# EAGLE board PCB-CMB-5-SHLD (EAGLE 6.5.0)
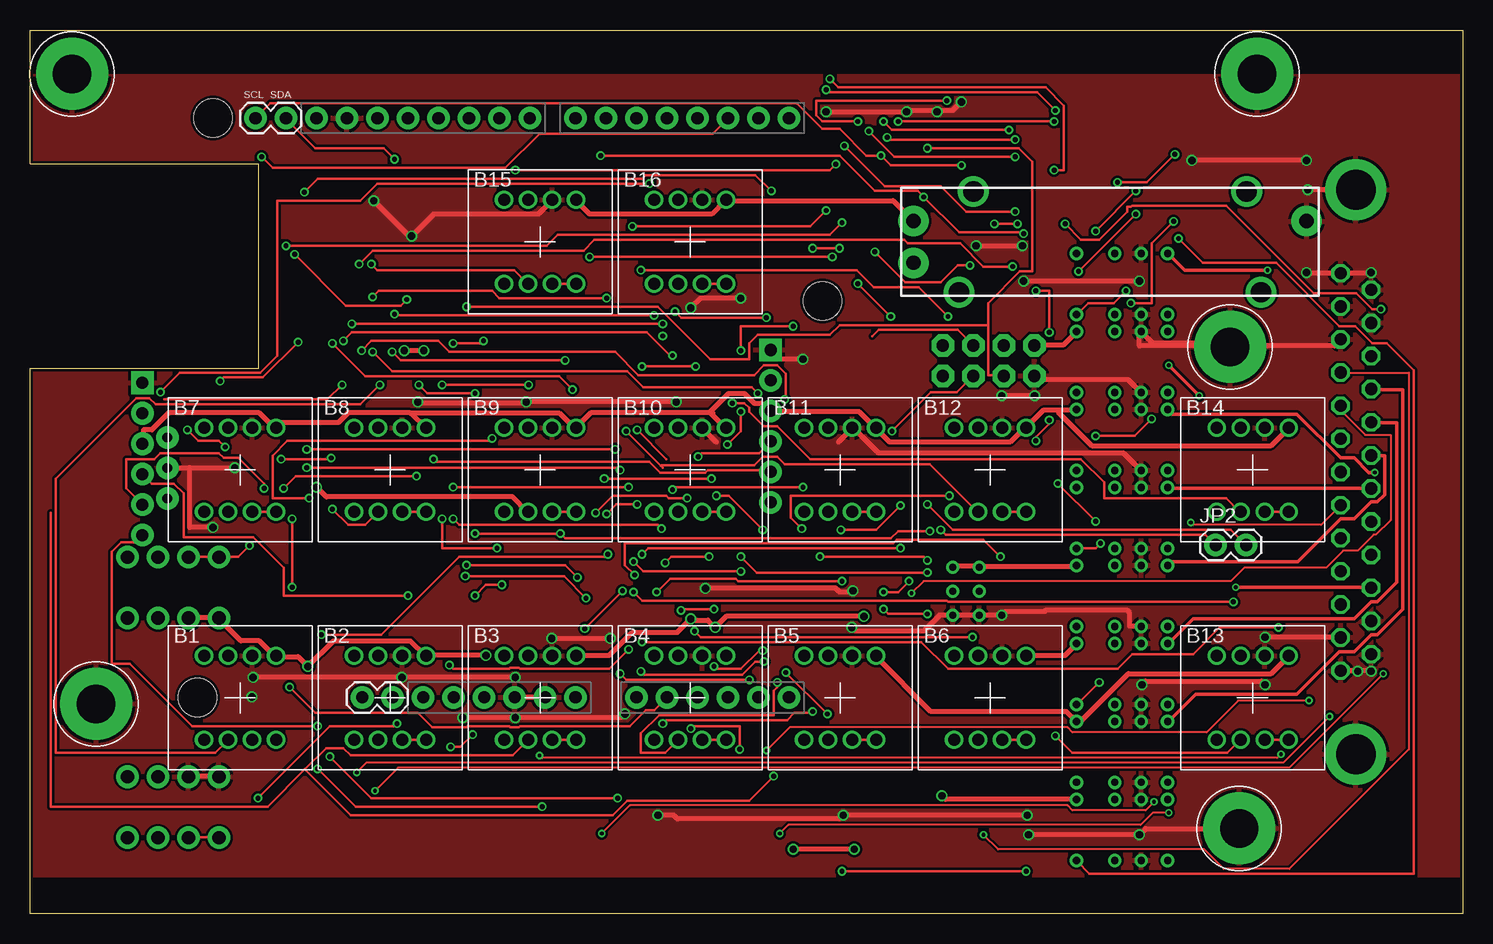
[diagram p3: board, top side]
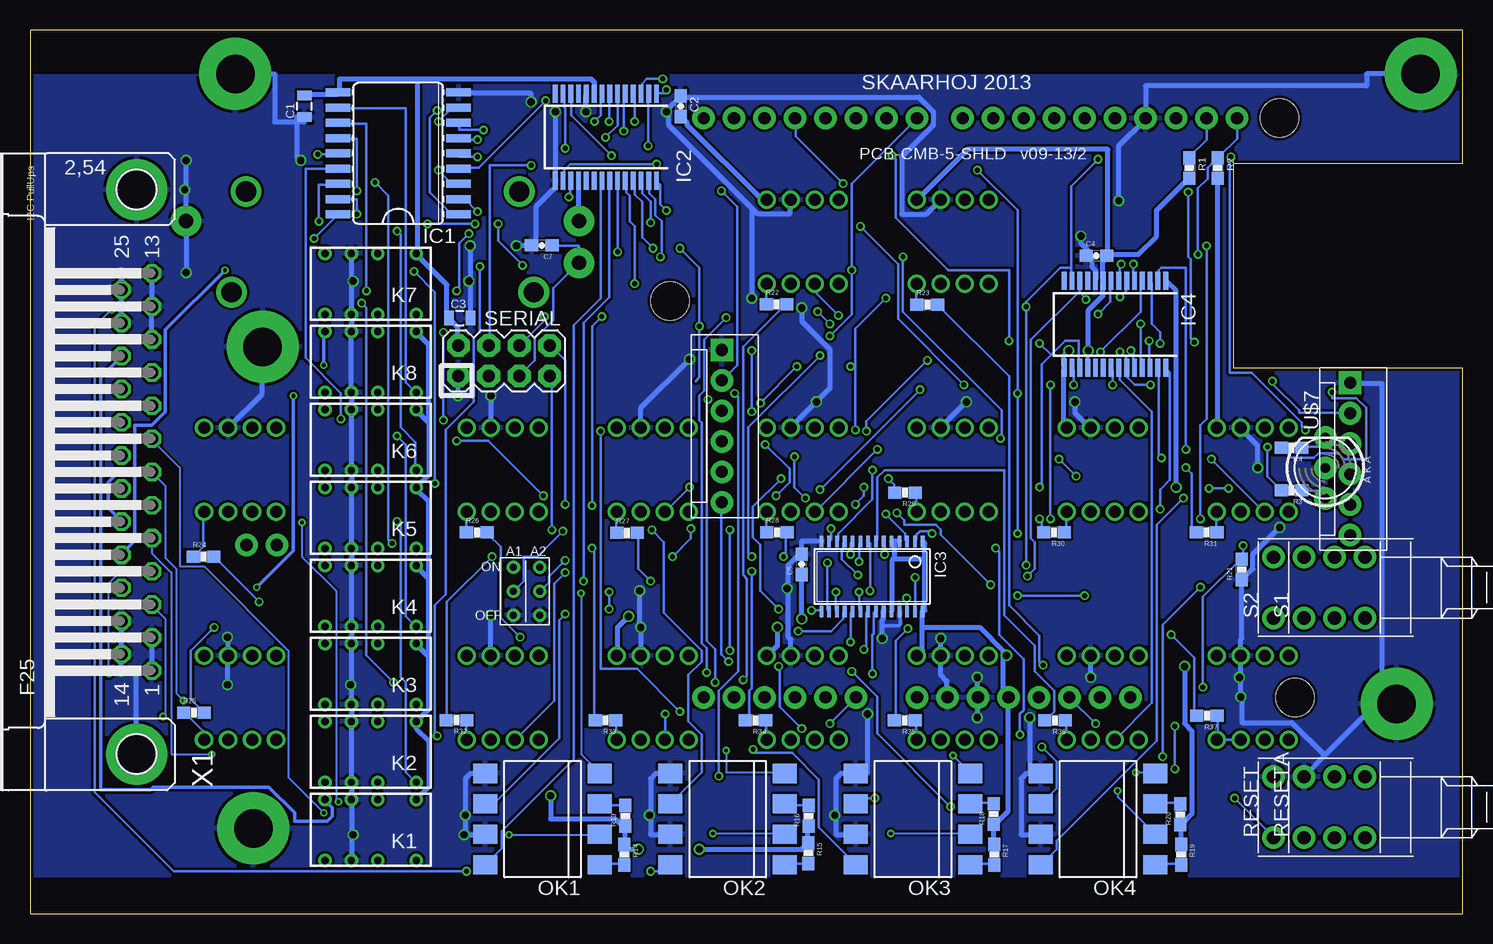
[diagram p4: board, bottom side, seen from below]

Size 119.38 x 73.66 mm. Coordinates in mm from the lower left corner, seen from the top.
Outline: 0,0 0,45.47 19.05,45.47 19.05,62.5 0,62.5 0,73.66 119.38,73.66 119.38,0 0,0
Copper layers (1*16): Top 0.035mm / dielectric 1.5mm / Bottom 0.035mm
Design rules "Fusion_eagle_rule_v1.1": minimum track width 6mil, minimum drill 12mil, track to track 6mil, track to pad 6mil, pad to pad 6mil, via to via 6mil, smd to smd 0mil, copper to edge 10mil, drill to drill 10mil, minimum pad ring 10mil, minimum via ring 6mil, stop-mask expansion 2mil, vias tented up to drill 100mil, thermal gap 10mil
Net classes: 0 default: width 0.203 mm, drill 0.406 mm, clearance 0.203 mm; 1 PWR: width 0.406 mm, drill 0.61 mm, clearance 0.203 mm; 2 RELAY LINES: width 0.305 mm, clearance 0.203 mm; 3 INput lines: clearance 0.203 mm
Holes 3.2 mm at 66.04,51.07 15.24,66.31 13.97,18.05
tRestrict: area 0,0 to 120,3; area 0,70 to 120,74
bRestrict: area 0,70 to 120,74; area 0,0 to 120,3

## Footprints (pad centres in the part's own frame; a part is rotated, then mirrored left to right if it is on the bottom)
NKK-NP01 = drill 1: 1 1,3.5; 2 -1,-3.5; L1 3,-3.5; L2 1,-3.5; L3 -1,3.5; L4 -3,3.5; LC1 3,3.5; LC2 -3,-3.5
0805 = smd 0.8 x 1.2: 1 -0.9,0; 2 0.9,0
0603-CAP = smd 1.1 x 1: 1 -0.85,0; 2 0.85,0
DUEMILANOVE_VIAS = drill 1.016 pad 1.88: 3.3V 50.8,13.97; 5V 50.8,16.51; A0 50.8,29.21; A1 50.8,31.75; A2 50.8,34.29; A3 50.8,36.83; A4 50.8,39.37; A5 50.8,41.91; AREF 2.54,2.54; D2 2.54,36.83; D3 2.54,34.29; D4 2.54,31.75; D5 2.54,29.21; D6 2.54,26.67; D7 2.54,24.13; D8 2.54,20.32; D9 2.54,17.78; D10 2.54,15.24; D11 2.54,12.7; D12 2.54,10.16; D13 2.54,7.62; GND@0 50.8,19.05; GND@1 50.8,21.59; GND@2 2.54,5.08; RES 50.8,11.43; RX 2.54,41.91; TX 2.54,39.37; VIN 50.8,24.13
SO18W = smd 0.66 x 2.032: 1 -5.08,-5.029; 2 -3.81,-5.029; 3 -2.54,-5.029; 4 -1.27,-5.029; 5 0,-5.029; 6 1.27,-5.029; 7 2.54,-5.029; 8 3.81,-5.029; 9 5.08,-5.029; 10 5.08,5.029; 11 3.81,5.029; 12 2.54,5.029; 13 1.27,5.029; 14 0,5.029; 15 -1.27,5.029; 16 -2.54,5.029; 17 -3.81,5.029; 18 -5.08,5.029
SSOP28 = smd 0.4 x 1.5: 1 -4.225,-3.625; 2 -3.575,-3.625; 3 -2.925,-3.625; 4 -2.275,-3.625; 5 -1.625,-3.625; 6 -0.975,-3.625; 7 -0.325,-3.625; 8 0.325,-3.625; 9 0.975,-3.625; 10 1.625,-3.625; 11 2.275,-3.625; 12 2.925,-3.625; 13 3.575,-3.625; 14 4.225,-3.625; 15 4.225,3.625; 16 3.575,3.625; 17 2.925,3.625; 18 2.275,3.625; 19 1.625,3.625; 20 0.975,3.625; 21 0.325,3.625; 22 -0.325,3.625; 23 -0.975,3.625; 24 -1.625,3.625; 25 -2.275,3.625; 26 -2.925,3.625; 27 -3.575,3.625; 28 -4.225,3.625
TSSOP28 = smd 0.305 x 0.991: 1 -4.225,-2.918; 2 -3.575,-2.918; 3 -2.925,-2.918; 4 -2.275,-2.918; 5 -1.625,-2.918; 6 -0.975,-2.918; 7 -0.325,-2.918; 8 0.325,-2.918; 9 0.975,-2.918; 10 1.625,-2.918; 11 2.275,-2.918; 12 2.925,-2.918; 13 3.575,-2.918; 14 4.225,-2.918; 15 4.225,2.918; 16 3.575,2.918; 17 2.925,2.918; 18 2.275,2.918; 19 1.625,2.918; 20 0.975,2.918; 21 0.325,2.918; 22 -0.325,2.918; 23 -0.975,2.918; 24 -1.625,2.918; 25 -2.275,2.918; 26 -2.925,2.918; 27 -3.575,2.918; 28 -4.225,2.918
1X02 = drill 1.016 pad 1.88: 1 0,0; 2 2.54,0
MOLEX-1X6 = drill 1.016 pad 1.88 square: 1 0,0 | drill 1.016 pad 1.88: 2 2.54,0; 3 5.08,0; 4 7.62,0; 5 10.16,0; 6 12.7,0
DS2Y = drill 0.6: 1 1.2,0.46; 16 1.2,5.54; O1 4.4,0.46; O2 4.4,5.54; P1 6.6,0.46; P2 6.6,5.54; S1 8.8,0.46; S2 8.8,5.54
DIL8-SMD = smd 1.6 x 2: 1 -3.81,-4.77; 2 -1.27,-4.77; 3 1.27,-4.77; 4 3.81,-4.77; 5 3.81,4.77; 6 1.27,4.77; 7 -1.27,4.77; 8 -3.81,4.77
SLIDER20 = drill 1.194 pad 2.54: 1 -16.383,1.74; 2A -16.383,-1.74; 3 16.383,1.74 | drill 1.702: P$1 -11.392,4.191; P$2 11.392,4.191; P$3 12.598,-4.191; P$4 -12.598,-4.191
0603-RES = smd 1.1 x 1: 1 -0.85,0; 2 0.85,0
PUSHBUTTON = drill 1.1 pad 1.88: 1 2.54,2.54; 2 2.54,-2.54; 3 -2.54,2.54; 4 -2.54,-2.54
2X4 = drill 1.016 pad 1.88 octagon: 1 -3.81,-1.27; 2 -3.81,1.27; 3 -1.27,-1.27; 4 -1.27,1.27; 5 1.27,-1.27; 6 1.27,1.27; 7 3.81,-1.27; 8 3.81,1.27
3.2MMPAD6MM = drill 3.2 pad 6: P$1 0,0
LED5MM-BICOLOR = drill 0.813 pad 1.88: A2 2.54,0; A3 -2.54,0; K1 0,0
2BITADDR = drill 0.6: A1 0,0; A2 2.2,0; H2 0,2; H3 2.2,2; L2 0,-2; L3 2.2,-2
F25HP = drill 1.016 octagon: 1 -16.561,-1.27; 2 -13.792,-1.27; 3 -11.049,-1.27; 4 -8.28,-1.27; 5 -5.512,-1.27; 6 -2.769,-1.27; 7 0,-1.27; 8 2.769,-1.27; 9 5.512,-1.27; 10 8.28,-1.27; 11 11.049,-1.27; 12 13.792,-1.27; 13 16.561,-1.27; 14 -15.189,1.27; 15 -12.421,1.27; 16 -9.652,1.27; 17 -6.909,1.27; 18 -4.14,1.27; 19 -1.372,1.27; 20 1.372,1.27; 21 4.14,1.27; 22 6.909,1.27; 23 9.652,1.27; 24 12.421,1.27; 25 15.189,1.27 | drill 3.302 pad 5.08: G1 -23.52,0; G2 23.52,0

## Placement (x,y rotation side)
B1  NKK-NP01-SINGLECOLOR  [NKK-NP01]  17.5,18 0 top
B2  NKK-NP01-SINGLECOLOR  [NKK-NP01]  30,18 0 top
B3  NKK-NP01-SINGLECOLOR  [NKK-NP01]  42.5,18 0 top
B4  NKK-NP01-SINGLECOLOR  [NKK-NP01]  55,18 0 top
B5  NKK-NP01-SINGLECOLOR  [NKK-NP01]  67.5,18 0 top
B6  NKK-NP01-SINGLECOLOR  [NKK-NP01]  80,18 0 top
B7  NKK-NP01-SINGLECOLOR  [NKK-NP01]  17.5,37 0 top
B8  NKK-NP01-SINGLECOLOR  [NKK-NP01]  30,37 0 top
B9  NKK-NP01-SINGLECOLOR  [NKK-NP01]  42.5,37 0 top
B10  NKK-NP01-SINGLECOLOR  [NKK-NP01]  55,37 0 top
B11  NKK-NP01-SINGLECOLOR  [NKK-NP01]  67.5,37 0 top
B12  NKK-NP01-SINGLECOLOR  [NKK-NP01]  80,37 0 top
B13  NKK-NP01-SINGLECOLOR  [NKK-NP01]  101.88,18 0 top
B14  NKK-NP01-SINGLECOLOR  [NKK-NP01]  101.88,37 0 top
B15  NKK-NP01-SINGLECOLOR  [NKK-NP01]  42.5,56 0 top
B16  NKK-NP01-SINGLECOLOR  [NKK-NP01]  55,56 0 top
C1  100nF  [0805]  96.52,67.31 90 bottom
C2  100nF  [0603-CAP]  65.15,67.31 270 bottom
C3  10uF  [0805]  83.57,49.66 0 bottom
C4  100nF  [0603-CAP]  30.51,54.86 0 bottom
C5  100nF  [0603-CAP]  55.07,29.13 90 bottom
C7  10nF  [0603-CAP]  76.73,55.71 180 bottom
GND  ARDUINO_SHIELDNO_SILK  [DUEMILANOVE_VIAS]  21.34,68.85 270 top
IC1  ULN2803A  [SO18W]  88.7,63.38 90 bottom
IC2  MCP23017SS  [SSOP28]  71.39,64.73 180 bottom
IC3  PCA9685  [TSSOP28]  49.21,28.12 180 bottom
IC4  MCP23017SS  [SSOP28]  28.97,49.12 180 bottom
JP1  [1X02]  27.69,18.05 0 top
JP2  [1X02]  98.81,30.75 0 top
JP3  [MOLEX-1X6]  61.72,47 270 bottom
JP4  [1X02]  21.34,66.31 180 top
JP5  [MOLEX-1X6]  9.36,44.26 270 bottom
K1  RELAY5VIM03  [DS2Y]  86,10 180 bottom
K2  RELAY5VIM03  [DS2Y]  86,16.5 180 bottom
K3  RELAY5VIM03  [DS2Y]  86,23 180 bottom
K4  RELAY5VIM03  [DS2Y]  86,29.5 180 bottom
K5  RELAY5VIM03  [DS2Y]  86,36 180 bottom
K6  RELAY5VIM03  [DS2Y]  86,42.5 180 bottom
K7  RELAY5VIM03  [DS2Y]  86,55.5 180 bottom
K8  RELAY5VIM03  [DS2Y]  86,49 180 bottom
OK1  LTV826S  [DIL8-SMD]  76.67,7.9 90 bottom
OK2  LTV826S  [DIL8-SMD]  61.24,7.9 90 bottom
OK3  LTV826S  [DIL8-SMD]  45.81,7.9 90 bottom
OK4  LTV826S  [DIL8-SMD]  30.38,7.9 90 bottom
POT1  10K Linear  [SLIDER20]  90,56 0 top
R1  1K5  [0603-RES]  22.77,62.15 270 bottom
R2  1K5  [0603-RES]  20.4,62.15 270 bottom
R3  270  [0603-RES]  14.24,35.29 180 bottom
R4  270  [0603-RES]  14.24,38.83 180 bottom
R13  330R  [0603-RES]  69.76,8.18 90 bottom
R14  330R  [0603-RES]  69.86,4.93 270 bottom
R15  330R  [0603-RES]  54.53,5.06 270 bottom
R16  330R  [0603-RES]  54.47,8.18 90 bottom
R17  330R  [0603-RES]  39.03,4.93 270 bottom
R18  330R  [0603-RES]  39.06,8.32 90 bottom
R19  330R  [0603-RES]  23.46,4.93 270 bottom
R20  330R  [0603-RES]  23.52,8.3 90 bottom
R21  10K  [0603-RES]  18.41,28.72 90 bottom
R22  100R  [0603-RES]  57.16,50.8 0 bottom
R23  100R  [0603-RES]  44.61,50.77 0 bottom
R24  100R  [0603-RES]  104.91,29.77 0 bottom
R25  100R  [0603-RES]  105.72,16.77 0 bottom
R26  100R  [0603-RES]  82.15,31.79 0 bottom
R27  100R  [0603-RES]  69.62,31.75 0 bottom
R28  100R  [0603-RES]  57.14,31.82 0 bottom
R29  100R  [0603-RES]  46.47,35.11 180 bottom
R30  100R  [0603-RES]  34.04,31.8 180 bottom
R31  100R  [0603-RES]  21.32,31.8 180 bottom
R32  100R  [0603-RES]  83.84,16.16 180 bottom
R33  100R  [0603-RES]  71.41,16.14 180 bottom
R34  100R  [0603-RES]  58.93,16.12 180 bottom
R35  100R  [0603-RES]  46.48,16.12 180 bottom
R36  100R  [0603-RES]  33.96,16.12 180 bottom
R37  100R  [0603-RES]  21.31,16.5 180 bottom
RESET  [PUSHBUTTON]  13.21,8.89 90 bottom
RESETA  [PUSHBUTTON]  10.67,8.89 90 bottom
S1  [PUSHBUTTON]  10.67,27.19 90 bottom
S2  [PUSHBUTTON]  13.21,27.19 90 bottom
SERIAL  M04X2  [2X4]  79.88,46.1 0 bottom
U$4  GNDPAD6MM  [3.2MMPAD6MM]  100,47.25 0 top
U$7  LEDBICOLOR-AKA  [LED5MM-BICOLOR]  11.44,37.16 90 bottom
U$15  GNDPAD6MM  [3.2MMPAD6MM]  100.77,7.12 0 top
U$18  GNDPAD6MM  [3.2MMPAD6MM]  102.26,70 0 top
U$19  2BITADDR  [2BITADDR]  79.1,26.89 0 bottom
U$20  GNDPAD6MM  [3.2MMPAD6MM]  5.5,17.5 0 top
U$21  GNDPAD6MM  [3.2MMPAD6MM]  3.5,70 0 top
X1  DB25F  [F25HP]  110.49,36.83 90 bottom

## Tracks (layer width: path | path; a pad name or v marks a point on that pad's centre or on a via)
5V  (via drill 0.61)
  Top 0.406: B15.LC1 45.52,59.44 46.63,58.32 56.79,58.32 57.91,59.44 B16.LC1 58.12,59.44 71.93,59.44 73.56,57.81 POT1.1 | 56.69,41.76 46.74,41.76 45.52,40.54 B9.LC1 45.31,40.54 44.09,41.76 31.9,41.76 31.8,41.66 | 56.79,41.66 57.91,40.54 B10.LC1 | 56.79,41.66 56.69,41.76 | 56.9,41.76 56.79,41.66 | v32.82,46.94 v31.19,46.94 | 31.8,41.66 32.92,40.54 B8.LC1 | 31.8,41.66 31.7,41.76 26.52,41.76 25.7,40.95 20.93,40.95 20.52,40.54 B7.LC1 20.32,40.54 19.1,41.76 11.58,41.76 10.16,40.34 9.45,40.34 9.45,39.22 JP5.3 | S1.3 13.21,24.69 15.75,24.69 S2.3 15.85,24.49 17.58,22.76 19.1,22.76 20.32,21.54 B1.LC1 20.52,21.44 22.35,21.44 v23.16,20.62 25.3,22.76 31.7,22.76 32.92,21.54 B2.LC1 33.12,21.54 v38,21.54 | B3.LC1 45.52,21.54 48.26,21.54 50.19,23.47 53.95,23.47 v55.07,24.59 55.17,24.49 56.49,24.49 v57.1,23.88 58.01,24.79 v69.49,24.79 | K8.1 87.17,48.46 86.16,47.45 83.72,47.45 SERIAL.2 | 85.65,41.96 87.17,41.96 K6.1 | 85.65,41.96 84.43,41.96 83.01,40.54 B12.LC1 82.8,40.44 81.69,39.32 71.63,39.32 70.61,40.34 B11.LC1 70.41,40.54 69.09,41.86 61.77,41.86 JP3.3 61.57,41.96 60.96,42.57 60.35,42.57 59.54,43.38 58.22,43.38 56.69,41.86 56.69,41.76 | B14.LC1 104.85,40.44 103.43,39.01 88.49,39.01 85.65,41.86 85.65,41.96 | v68.68,5.38 v63.6,5.38 | U$19.H3 76.91,28.96 79.05,28.96 U$19.H2 79.25,28.96 87.17,28.96 K4.1 | K3.1 87.17,22.45 86.26,21.54 83.01,21.54 B6.LC1 | B5.LC1 70.51,21.44 75.08,16.87 86.36,16.87 87.17,16.05 K2.1 87.38,16.05 87.58,16.05 91.54,20.02 103.43,20.02 104.85,21.44 B13.LC1 | v76,9.86 76.3,9.55 87.17,9.55 K1.1
  Bottom 0.305: v31.19,46.94 31.25,46.94 IC4.18
  Bottom 0.406: IC2.18 73.66,61.06 73.66,57.81 POT1.1 | C2.2 65.13,66.45 64.62,65.94 64.62,65.73 58.42,59.54 58.01,59.54 B16.LC1 | R2.2 20.42,61.27 20.42,40.54 B7.LC1 | R1.2 22.86,61.27 25.5,58.62 25.5,56.49 27.03,54.97 29.57,54.97 29.57,54.86 C4.2 | B8.LC1 33.02,40.54 33.22,40.74 33.22,45.41 IC4.15 33.22,45.62 33.22,46.53 v32.82,46.94 | v31.19,46.94 31.19,50.29 29.97,51.51 29.97,52.73 IC4.9 29.97,52.93 29.97,54.36 29.67,54.66 C4.2 | B15.LC1 45.41,59.54 41.25,63.7 29.57,63.7 29.57,55.07 C4.2 | R19.1 23.47,5.79 23.47,7.42 R20.1 23.37,7.52 22.55,8.33 22.55,15.24 23.16,15.85 v23.16,20.62 | R17.1 39.12,5.79 39.12,7.42 R18.1 38.91,7.52 37.9,8.53 37.9,17.98 GND.5V 37.9,18.19 38.3,18.59 38.3,21.54 | 47.35,31.09 47.55,31.09 IC3.5 | 47.35,31.09 46.94,31.09 IC3.4 | 47.35,29.67 47.55,29.46 47.55,25.3 IC3.24 | 47.35,31.09 47.35,29.67 | 45.01,23.88 45.01,21.95 45.41,21.54 B3.LC1 | 45.01,23.88 45.01,25.2 IC3.28 44.81,25.3 44.81,29.57 | 44.81,29.57 44.81,30.89 44.91,30.99 IC3.1 | v55.07,24.59 55.07,28.25 C5.1 | v57.1,23.88 57.1,22.35 57.91,21.54 B4.LC1 | 44.81,29.57 47.24,29.57 47.35,29.67 | 38.3,21.54 38.3,21.95 40.23,23.88 45.01,23.88 | 38.3,21.54 v38,21.54 | C1.2 96.52,68.28 93.78,68.28 93.78,68.38 IC1.10 93.57,68.58 93.57,69.6 87.07,69.6 | 87.07,69.6 72.64,69.6 72.34,69.29 72.34,68.38 IC2.9 | SERIAL.2 83.72,47.45 83.72,48.87 84.43,49.58 C3.1 84.63,49.78 84.63,52.43 87.17,54.97 K7.1 87.07,55.17 87.07,69.6 | 86.26,41.05 87.17,41.96 K6.1 | 86.26,41.05 86.16,40.95 86.16,36.58 87.17,35.56 K5.1 87.17,35.36 86.16,34.34 86.16,28.14 86.26,28.04 | K8.1 87.17,48.46 86.16,47.45 86.16,41.15 86.26,41.05
  Bottom 0.406: R16.1 54.56,7.32 54.56,5.99 R15.1 54.66,5.79 55.07,5.38 v63.6,5.38 | v68.68,5.38 69.6,5.38 69.6,5.79 R14.1 69.8,5.79 69.8,7.32 R13.1 70,7.32 70.61,7.92 76,7.92 v76,9.86 | K1.1 87.17,9.55 86.16,10.57 86.16,14.43 87.17,15.44 87.17,15.95 K2.1 87.07,16.15 86.16,17.07 86.16,21.44 86.26,21.54 | 86.26,21.54 87.17,22.45 K3.1 | 86.26,28.04 86.16,27.94 86.16,21.64 86.26,21.54 | 86.26,28.04 87.17,28.96 K4.1 | v69.49,24.79 70.41,23.88 70.41,21.54 B5.LC1
A1  (via drill 0.41)
  Top 0.203: v74.98,31.9 72.34,31.9 71.73,31.29 44.6,31.29 v44.2,31.7 v37.08,31.7 | v32.41,44.09 33.12,43.38 v37.08,43.38 | v67.16,62.48 66.65,61.98 v40.44,61.98
  Bottom 0.203: v44.2,31.7 44.2,31.9 45.21,31.9 45.52,31.6 45.52,31.19 45.62,31.09 IC3.2 | v74.98,31.9 77.11,29.77 78.23,29.77 78.23,27.74 79.05,26.92 U$19.A1 | v32.41,44.09 32.41,45.31 32.51,45.41 IC4.16 | v37.08,31.7 v37.08,43.38 37.08,58.62 v40.44,61.98 | v67.16,62.48 74.37,62.48 74.88,61.98 74.88,61.16 IC2.16
A1CFG  (via drill 0.41)
  Top 0.203: v18.29,30.68 17.37,29.77 15.75,29.77 | v21.64,18.9 23.77,16.76 32.31,16.76 33.53,15.54 36.37,15.54 36.47,15.65 39.93,15.65 40.03,15.54 40.74,15.54 40.84,15.65 49.99,15.65 51.31,16.97 52.02,16.97 53.03,17.98 GND.A1 | 15.75,29.77 13.21,29.77 S1.1 | 15.75,29.77 S2.1
  Bottom 0.203: v18.29,30.68 18.29,29.77 18.39,29.67 R21.2 18.49,29.57 21.64,26.42 v21.64,18.9
A2  (via drill 0.41)
  Top 0.203: v48.06,33.33 48.87,34.14 v50.6,34.14 | v35.26,35.56 v49.89,35.56 | v47.55,63.2 67.46,63.2 70.41,60.25 73.97,60.25 v74.47,59.74 77.42,56.79 82.7,56.79 v82.8,56.69 | v37.8,47.75 37.59,47.55 v35.26,47.55 | v74.78,29.46 74.47,29.77 v65.84,29.77 | v64.31,32.11 63.4,33.02 63.4,34.85 v76.61,34.85 | v83.82,39.42 83.82,39.73 84.94,40.84 v84.94,41.15 | v84.94,48.46 84.94,51.92 v83.82,51.92
  Bottom 0.203: v48.06,33.33 46.43,31.7 46.43,31.19 46.33,31.09 IC3.3 | v50.6,34.14 49.89,34.85 v49.89,35.56 | v35.26,35.56 35.05,35.76 35.05,45.82 34.29,46.58 | 34.29,46.58 33.12,47.75 32,47.75 32,45.62 31.9,45.52 IC4.17 | v74.47,59.74 74.37,59.84 74.37,61.06 IC2.17 | v47.55,63.2 47.24,62.89 47.24,58.01 42.88,53.65 37.8,53.65 v37.8,47.75 | 34.29,46.58 v35.26,47.55 | v74.78,29.46 76.1,28.14 76.1,27.64 76.81,26.92 U$19.A2 | v65.84,29.77 64.31,31.29 v64.31,32.11 | v76.61,34.85 81.18,39.42 v83.82,39.42 | v84.94,48.46 v84.94,41.15 | v83.82,51.92 83.62,52.12 83.62,55.88 v82.8,56.69
D2  (via drill 0.41)
  Top 0.203: v16.26,38.91 15.75,39.42 14.02,39.42 v13.11,40.34 | v19.3,63.09 20.22,62.18 39.62,62.18 42.47,65.02 56.9,65.02 58.12,66.24 GND.D2
  Bottom 0.203: v16.26,38.91 16.26,36.47 15.14,35.36 R3.2 | v13.11,40.34 13.41,40.64 13.41,40.95 17.58,45.11 19.41,45.11 19.41,62.99 v19.3,63.09
D3  (via drill 0.41)
  Top 0.203: v10.87,43.48 12.5,45.11 19.2,45.11 20.62,46.53 20.62,59.44 27.53,59.44 28.96,60.86 v51.61,60.86
  Bottom 0.203: v10.87,43.48 10.87,42.98 8.84,42.98 8.03,42.16 8.03,37.9 9.86,37.9 10.36,38.41 11.99,38.41 12.39,38 14.22,38 15.04,38.81 R4.2 | v51.61,60.86 55.58,64.82 55.58,66.24 GND.D3
DISP_DATA_OUT  (via drill 0.41)
  Top 0.203: 70.21,48.16 70.71,48.67 77.32,48.67 78.54,47.45 SERIAL.6 | v76.5,49.78 74.07,52.22 70.31,52.22 68.89,53.65 v50.9,53.65
  Bottom 0.203: v52.73,48.16 50.9,49.99 v50.9,53.65 50.9,60.86 45.52,66.24 GND.D7 | v76.5,49.78 76.5,49.48 78.54,47.45 SERIAL.6
GND  (via drill 0.61)
  Top 0.406: RESETA.1 13.21,11.48 15.75,11.48 RESET.1 | v111.76,53.44 109.22,53.44 X1.13 109.12,53.44 v106.38,53.44 | v106.38,62.79 v96.83,62.79 | X1.G2 v106.48,60.35 | v68.48,23.88 68.78,23.57 74.47,23.57 75.79,24.89 76.71,24.89 U$19.L3 76.91,24.89 79.05,24.89 U$19.L2 79.25,24.89 v80.97,24.89 81.28,25.2 84.53,25.2 84.63,25.3 91.44,25.3 91.64,25.09 91.64,23.98 92.56,23.98 K4.P2 | v56.29,27.13 67.16,27.13 67.46,26.82 68.48,26.82 v68.58,26.92 | v78.84,55.68 v82.7,55.68 | v43.48,22.96 v48.36,22.96 | v40.44,19.71 v30.99,19.71 v18.59,19.71 | GND.GND@1 42.88,18.09 40.44,18.09 GND.GND@0 | v36.07,16.36 v40.44,16.36 49.28,16.36 v49.58,16.66 | v102.92,23.06 109.22,23.06 X1.2 | v111.76,20.22 111.66,20.32 110.64,20.32 | 110.64,20.32 109.22,20.32 X1.1 | v110.64,20.22 110.64,20.32 | v52.32,8.23 53.65,8.23 53.95,7.92 67.46,7.92 v67.77,8.23 v83.11,8.23 | v83.72,43.18 v80.97,43.18 | v83.21,6.6 v92.46,6.6 92.96,7.11 100.69,7.11 U$15.P$1 | v102.92,19.1 102.62,19.41 92.96,19.41 v92.66,19.1 | v92.46,52.73 v82.8,52.73 | v32.31,42.67 32.41,42.57 41.25,42.57 v41.35,42.67 v53.85,42.67 | 57.2,39.32 56.08,40.44 B10.1 | 67.36,39.32 68.48,40.44 B11.1 68.68,40.44 70.71,38.41 91.14,38.41 92.56,36.98 K6.P2 | B15.1 43.48,59.44 42.37,58.32 33.63,58.32 v31.8,56.49 31.7,56.59 31.5,56.59 v28.65,59.44 | v66.34,66.85 v73.05,66.85 73.15,66.95 75.59,66.95 | v77.62,67.67 76.91,66.95 75.59,66.95 | v75.59,66.85 75.59,66.95 | v64.41,46.23 62.48,46.23 61.77,46.94 JP3.1 | v55.07,50.49 55.88,51.31 v59.23,51.31 | SERIAL.1 83.72,44.81 84.02,44.5 91.54,44.5 92.56,43.48 K8.P2 | U$4.P$1 99.97,47.95 99.57,47.55 93.57,47.55 92.66,48.46 K8.P1 92.56,48.46 92.46,48.36 92.46,47.35 108.71,47.35 109.22,47.85 X1.11
  Top 0.406: 13.31,37.19 11.48,37.19 U$7.K1 | 13.31,37.19 v17.07,37.19 | 13.31,37.19 13.31,32.21 v15.24,32.21
  Bottom 0.305: IC3.25 46.86,25.2 46.86,24.14 47,24 48.36,24
  Bottom 0.406: IC4.10 30.58,52.83 30.58,53.65 30.89,53.95 30.89,54.76 31.09,54.97 C4.1 31.09,55.17 31.8,55.88 v31.8,56.49 | 18.49,19.71 v18.49,18.09 18.39,17.98 18.39,15.95 14.22,15.95 11.48,13.21 | 18.49,19.71 18.49,21.34 B1.1 18.49,21.54 18.49,22.86 18.39,22.96 18.39,27.84 R21.1 18.29,27.94 17.48,28.75 17.48,29.97 v15.24,32.21 | X1.24 X1.25 v111.76,53.44 | X1.13 X1.12 X1.11 | v96.83,62.79 97.13,63.09 97.13,66.45 96.52,66.45 C1.1 96.52,66 99,66 99,70 U$18.P$1 | 106.38,60.35 106.38,57.81 POT1.3 106.38,57.61 v106.38,53.44 | 106.38,60.35 v106.38,62.79 | v106.48,60.35 106.38,60.35 | IC3.14 53.44,31.09 55.07,31.09 55.07,30.07 C5.2 55.27,29.97 56.19,29.06 56.19,27.13 | 56.19,27.13 56.19,23.06 55.98,22.86 55.98,21.54 B4.1 | v80.97,24.89 80.97,21.54 B6.1 | B5.1 68.48,21.54 v68.48,23.88 68.58,23.98 v68.58,26.92 | v56.29,27.13 56.19,27.13 | v82.7,55.68 82.7,52.73 | 82.7,52.73 82.7,49.68 C3.2 | v78.84,55.68 77.72,55.68 C7.2 77.52,55.68 77.22,55.68 77.22,58.93 75.59,60.55 75.59,61.06 IC2.15 75.59,61.27 v75.59,66.85 | v48.36,22.96 48.36,24 48.36,24.49 48.26,24.59 48.26,25.2 IC3.23 | v43.48,22.96 43.48,21.54 B3.1 43.48,21.34 43.48,19.91 42.98,19.41 42.98,18.09 GND.GND@1 | OK4.7 35.15,6.6 36.78,6.6 36.78,11.28 36.37,11.68 35.15,11.68 OK4.5 36.07,11.79 v36.07,16.36 | v30.99,19.71 30.99,21.44 B2.1 | v40.44,19.71 40.44,18.09 GND.GND@0 40.44,17.88 v40.44,16.36 | X1.15 X1.14 v111.76,20.22 | v102.92,23.06 102.92,21.54 B13.1 102.92,21.34 v102.92,19.1 | X1.2 X1.1 | v110.64,20.22 110.54,20.12 110.54,13.31 X1.G1 | 52.22,8.23 52.22,11.28 51.82,11.68 50.6,11.68 OK3.5 50.39,11.68 49.68,11.68 49.58,11.79 v49.58,16.66
  Bottom 0.406: 52.22,8.23 52.22,6.6 50.6,6.6 OK3.7 | 67.67,8.23 67.67,11.28 67.26,11.68 66.04,11.68 OK2.5 | 67.67,8.23 67.67,6.6 66.04,6.6 OK2.7 | v52.32,8.23 52.22,8.23 | v67.77,8.23 67.67,8.23 | v80.97,43.18 80.97,40.54 B12.1 | v83.72,43.18 83.72,44.81 SERIAL.1 | 92.56,52.73 92.56,50.09 K7.P2 92.56,49.89 92.56,48.56 K8.P1 92.66,48.36 92.66,43.59 K8.P2 92.56,43.38 92.56,42.06 K6.P1 92.56,41.86 92.56,37.08 K6.P2 92.56,36.88 92.56,35.56 K5.P1 92.56,35.36 92.56,30.58 K5.P2 92.56,30.38 92.56,29.06 K4.P1 92.56,28.85 92.56,24.08 K4.P2 92.56,23.88 92.56,22.55 K3.P1 92.56,22.35 92.56,19.1 | 92.56,52.73 92.56,54.97 K7.P1 | 83.11,6.6 81.48,6.6 OK1.7 | 83.11,6.6 v83.11,8.23 83.11,11.28 82.7,11.68 81.48,11.68 OK1.5 | 92.56,6.6 92.56,9.35 K1.P1 92.56,9.55 92.56,10.87 K2.P2 92.56,11.07 92.56,15.85 K2.P1 92.56,16.05 92.56,17.37 K3.P2 92.56,17.58 92.56,19.1 | 92.56,6.6 92.56,4.47 K1.P2 | v83.21,6.6 83.11,6.6 | v92.46,6.6 92.56,6.6 | v92.66,19.1 92.56,19.1 | v82.8,52.73 82.7,52.73 | v92.46,52.73 92.56,52.73 | v18.59,19.71 18.49,19.71 | 11.48,13.21 7.21,17.48 5.59,17.48 U$20.P$1 6.71,17.58 6.71,44.2 9.35,44.2 JP5.1 | 11.48,13.21 13.21,11.48 RESETA.1 | v32.31,42.67 32.31,41.76 31.09,40.54 B8.1 | v41.35,42.67 43.48,40.54 B9.1 | B10.1 55.98,40.54 v53.85,42.67 52.73,43.79 52.73,47.04 55.07,49.38 v55.07,50.49 | v28.65,59.44 28.65,64.01 26.42,66.24 GND.GND@2 26.42,69 8,69 8,70 U$21.P$1 | 66.14,66.85 66.14,65.73 59.13,58.73 | 66.14,66.85 66.14,67.16 65.23,68.07 C2.1 65.02,68.07 45.31,68.07 44.09,66.85 44.09,65.73 46.74,63.09 46.74,58.32 44.7,58.32 43.59,59.44 B15.1 | 59.13,58.73 58.73,58.32 56.08,58.32 56.08,59.44 B16.1
  Bottom 0.406: v73.05,66.85 73.05,68.28 IC2.10 | v66.34,66.85 66.14,66.85 | v77.62,67.67 77.62,68.38 83.62,68.38 IC1.9 | v64.41,46.23 68.48,42.16 68.48,40.54 B11.1 | v59.23,51.31 59.23,58.62 59.13,58.73 | B14.1 102.82,40.54 100.08,43.28 100.08,47.95 U$4.P$1 | v17.07,37.19 17.07,39.01 18.49,40.44 B7.1
  pour Bottom: 0,0 120,0 120,74 0,74
  pour Top: 0,0 120,0 120,74 0,74
GPA0  (via drill 0.41)
  Top 0.203: v29.16,44.09 27.53,42.47 10.46,42.47 9.96,42.98 8.84,42.98 2.13,36.27 2.13,13.41 15.44,13.41 16.46,14.43 B1.2
  Bottom 0.203: v29.16,44.09 29.16,45.31 29.26,45.41 IC4.21
GPA1
  Bottom 0.203: IC4.22 28.55,45.41 28.55,44.5 25.91,41.86 25.91,17.58 28.96,14.53 B2.2
GPA2  (via drill 0.41)
  Top 0.203: v26.01,44.09 24.79,42.88 11.18,42.88 | 1.73,33.43 1.73,8.94 19.81,8.94 22.91,12.04 | 22.91,12.04 24.69,13.82 26.11,13.82 26.72,13.21 40.23,13.21 41.45,14.43 B3.2 | v28.55,46.84 30.18,45.21 49.78,45.21 51.1,43.89 60.15,43.89 v60.66,43.38 | v61.98,11.48 59.94,9.45 49.78,9.45 48.56,8.23 26.72,8.23 22.91,12.04
  Bottom 0.203: v26.01,44.09 27.33,44.09 27.94,44.7 27.94,45.41 IC4.23 28.04,45.52 28.04,46.33 v28.55,46.84 | v60.66,43.38 60.35,43.08 60.35,20.22 61.98,18.59 v61.98,11.48
GPA3  (via drill 0.41)
  Top 0.203: v27.64,46.94 28.45,47.75 34.04,47.75 34.95,46.84 48.77,46.84 50.7,44.91 60.35,44.91 61.16,45.72 62.28,45.72 62.99,45.01 62.99,42.88 v62.89,42.88 | v62.28,19.3 62.28,18.9 61.98,18.59 61.98,16.56 52.43,16.56 50.9,15.04 50.9,13.41 52.93,13.41 53.95,14.43 B4.2
  Bottom 0.203: v27.64,46.94 27.43,46.74 27.43,45.52 IC4.24 | v62.89,42.88 62.99,42.77 62.99,22.76 62.28,22.05 v62.28,19.3
GPA4  (via drill 0.41)
  Top 0.203: v52.73,49.17 v26.82,49.17 | v53.75,50.19 54.25,49.68 v61.37,49.68 | v66.45,16.66 v62.99,20.12
  Bottom 0.203: v26.82,49.17 26.82,45.62 26.72,45.52 IC4.25 | v53.75,50.19 v52.73,49.17 | v61.37,49.68 63.2,47.85 63.2,43.59 63.6,43.18 63.6,41.15 63.4,40.95 63.4,22.55 62.99,22.15 v62.99,20.12 | v66.45,16.66 66.45,14.53 B5.2
GPA5  (via drill 0.41)
  Top 0.203: v26.11,47.75 26.82,48.46 51.41,48.46 53.34,46.53 v53.54,46.53 | v59.23,29.77 60.55,28.45 v74.78,28.45
  Bottom 0.203: v26.11,47.75 26.11,45.52 IC4.26 | v53.54,46.53 59.54,40.54 59.54,30.07 v59.23,29.77 | v74.78,28.45 75.69,27.53 75.69,17.78 78.94,14.53 B6.2
GPA6  (via drill 0.41)
  Top 0.203: v25.09,38 24.99,37.9 v20.93,37.9
  Bottom 0.203: v25.09,38 25.3,38.2 25.3,45.41 IC4.27 | v20.93,37.9 16.56,33.53 B7.2
GPA7  (via drill 0.41)
  Top 0.203: v25.2,33.73 26.52,32.41 27.94,32.41 28.96,33.43 B8.2
  Bottom 0.203: v25.2,33.73 25.2,35.36 24.38,36.17 24.38,45.11 24.69,45.41 IC4.28
GPB0  (via drill 0.61)
  Top 0.406: v23.88,35.56 24.69,34.75 40.23,34.75 41.45,33.53 B9.2
  Bottom 0.406: v23.88,35.56 23.88,51.92 24.69,52.73 IC4.1
GPB1  (via drill 0.41)
  Top 0.203: v48.77,38.71 v23.06,38.71
  Bottom 0.203: v23.06,38.71 23.06,53.85 25.09,53.85 25.3,53.65 25.3,52.83 IC4.2 | v48.77,38.71 53.95,33.53 B10.2
GPB2  (via drill 0.41)
  Top 0.203: v25.2,47.55 27.94,44.81 44.09,44.81 v45.21,43.69 | 53.65,35.26 v53.54,35.36 53.65,35.36 53.85,35.56 v64.41,35.56 | 66.45,33.53 B11.2
  Bottom 0.203: v25.2,47.55 25.2,48.46 25.91,49.17 25.91,52.63 26.01,52.73 IC4.3 | v53.54,35.36 v45.21,43.69 | v64.41,35.56 66.45,33.53 B11.2
GPB3  (via drill 0.41)
  Top 0.203: v30.18,46.84 30.89,46.13 v44.6,46.13 | 52.73,37.19 52.58,37.34 | 52.58,37.34 v49.68,40.23 | B12.2 78.94,33.53 74.98,37.49 62.89,37.49 62.28,38.1 61.06,38.1 60.35,37.39 52.63,37.39 52.58,37.34
  Bottom 0.203: v30.18,46.84 26.82,50.19 26.82,52.63 26.72,52.73 IC4.4 | v44.6,46.13 49.68,41.05 v49.68,40.23
GPB4  (via drill 0.41)
  Top 0.203: v27.43,54.15 28.55,55.27 46.13,55.27 47.04,56.19 72.85,56.19 73.15,55.88 77.52,55.88 79.45,53.95 v81.89,53.95 | v85.45,14.83 86.87,13.41 99.77,13.41 100.79,14.43 B13.2
  Bottom 0.203: v27.43,54.15 27.43,52.83 IC4.5 | v81.89,53.95 81.89,48.46 82.4,47.95 82.4,42.67 84.73,40.34 84.73,26.62 85.65,25.7 85.65,15.04 v85.45,14.83
GPB5  (via drill 0.41)
  Top 0.203: v28.55,51.41 29.06,51.92 38.51,51.92 39.12,51.31 v48.06,51.31 | 53.03,37.9 v50.6,40.34 | B14.2 100.79,33.53 99.67,34.65 89.51,34.65 89.51,35.97 87.58,37.9 65.02,37.9 62.28,40.64 61.16,40.64 59.94,41.86 59.94,42.16 59.54,42.57 v58.52,42.57 | v51,45.62 v55.47,45.62
  Bottom 0.203: v28.55,51.41 28.04,51.92 28.04,52.73 IC4.6 | v48.06,51.31 50.6,48.77 50.6,45.62 | v50.6,40.34 50.6,45.62 | v55.47,45.62 v58.52,42.57 | 50.6,45.62 v51,45.62
GPB6  (via drill 0.41)
  Top 0.203: v28.45,54.15 28.96,53.65 40.34,53.65 41.45,52.53 B15.2
  Bottom 0.203: v28.45,54.15 28.55,54.05 28.55,52.83 IC4.7
GPB7  (via drill 0.41)
  Top 0.203: v30.38,49.99 30.48,49.89 v52.02,49.89
  Bottom 0.203: v30.38,49.99 29.36,51 29.36,52.73 IC4.8 | v52.02,49.89 53.95,51.82 53.95,52.43 B16.2
I2C_SCL  (via drill 0.41)
  Top 0.203: v46.33,26.31 44.5,28.14 v36.27,28.14 | v77.62,62.38 71.73,62.38 v70.92,63.2 69.7,63.2 67.46,65.43 66.04,65.43 63.91,67.56 20.02,67.56 18.8,66.34 JP4.2 | v31.39,51.21 30.89,50.7 26.31,50.7 v22.05,54.97
  Bottom 0.203: v46.33,26.31 46.33,25.3 IC3.26 | v36.27,28.14 35.66,28.75 35.66,30.99 35.97,31.29 35.97,47.85 31.95,51.87 | 31.95,51.87 31.9,51.92 31.9,52.73 IC4.12 | JP4.2 18.8,64.62 20.32,63.09 R2.1 20.42,62.99 21.23,62.18 21.23,61.27 22.05,60.45 v22.05,54.97 | v70.92,63.2 74.27,66.55 74.27,68.28 IC2.12 | v77.62,62.38 81.08,62.38 81.08,47.45 SERIAL.4 | 31.95,51.87 31.39,51.31 v31.39,51.21
I2C_SDA  (via drill 0.41)
  Top 0.203: v74.78,63.8 82.4,63.8 83.52,62.69 83.52,53.54 82.5,53.54 79.86,50.9 79.86,49.07 | 79.86,49.07 79.86,44.91 81.08,44.91 SERIAL.3 | v45.62,28.04 44.6,29.06 v36.37,29.06 | v30.38,62.89 29.46,63.8 23.77,63.8 21.34,66.24 JP4.1 | 79.86,49.07 67.46,49.07 66.65,48.26 60.66,48.26 59.94,47.55 59.94,46.23 56.69,46.23 52.32,50.6 v36.37,50.6
  Bottom 0.203: v74.78,63.8 74.78,67.16 74.88,67.26 74.88,68.28 IC2.13 | JP4.1 21.34,64.52 22.76,63.09 R1.1 | v45.62,28.04 45.62,25.3 IC3.27 | v36.37,29.06 v36.37,50.6 36.37,51 33.53,53.85 32.61,53.85 | 32.61,53.85 32.61,52.83 IC4.13 | v30.38,62.89 32.61,60.66 32.61,53.85
L0
  Bottom 0.203: R37.1 20.42,16.46 20.42,14.53 B1.L1 20.32,14.53 18.59,14.53 B1.L2
L1
  Top 0.203: B2.L2 31.09,14.53 32.92,14.53 B2.L1
  Bottom 0.203: R36.1 33.02,16.05 33.02,14.53 B2.L1
L2
  Top 0.203: B3.L2 43.59,14.53 45.41,14.53 B3.L1
  Bottom 0.203: R35.1 45.62,16.05 45.52,15.95 45.52,14.53 B3.L1
L3
  Top 0.203: B4.L2 56.08,14.53 57.91,14.53 B4.L1
  Bottom 0.203: R34.1 58.01,16.05 58.01,14.53 B4.L1
L4
  Top 0.203: B5.L2 68.58,14.53 70.41,14.53 B5.L1
  Bottom 0.203: R33.1 70.51,16.05 70.51,14.53 B5.L1
L5
  Top 0.203: B6.L2 81.08,14.53 82.91,14.53 B6.L1
  Bottom 0.203: R32.1 83.01,16.15 83.01,14.53 B6.L1
L6
  Top 0.203: B7.L2 18.59,33.53 20.42,33.53 B7.L1
  Bottom 0.203: R31.1 20.52,31.8 20.52,33.43 B7.L1
L7
  Top 0.203: B8.L2 31.09,33.53 32.92,33.53 B8.L1
  Bottom 0.203: R30.1 33.12,31.8 33.02,31.9 33.02,33.43 B8.L1
L8
  Top 0.203: B9.L2 43.59,33.53 45.41,33.53 B9.L1
  Bottom 0.203: R29.1 45.62,35.05 45.52,34.95 45.52,33.53 B9.L1
L9
  Top 0.203: B10.L2 56.08,33.53 57.91,33.53 B10.L1
  Bottom 0.203: R28.1 58.01,31.9 58.01,33.43 B10.L1
L10
  Top 0.203: B11.L2 68.58,33.53 70.41,33.53 B11.L1
  Bottom 0.203: R27.1 70.51,31.8 70.51,33.43 B11.L1
L11
  Top 0.203: B12.L2 81.08,33.53 82.91,33.53 B12.L1
  Bottom 0.203: R26.1 83.01,33.43 B12.L1
L12
  Top 0.203: B13.L2 102.92,14.53 104.85,14.53 B13.L1
  Bottom 0.203: R25.1 106.48,16.76 104.95,15.24 104.95,14.53 B13.L1
L13
  Top 0.203: B14.L2 102.92,33.53 104.85,33.53 B14.L1
  Bottom 0.203: R24.1 105.66,29.87 104.95,30.58 104.95,33.43 B14.L1
L14
  Top 0.203: B15.L2 43.59,52.53 45.41,52.53 B15.L1
  Bottom 0.203: R23.1 45.52,50.8 45.52,52.43 B15.L1
L15
  Top 0.203: B16.L2 56.08,52.53 57.91,52.53 B16.L1
  Bottom 0.203: R22.1 58.01,50.9 58.01,52.43 B16.L1
N$1
  Bottom 0.305: K1.S1 94.79,9.45 94.18,8.84 94.18,8.13 94.59,7.72 97.33,7.72 97.33,8.43 99.47,10.57 109.12,10.57 109.32,10.36 113.49,10.36 113.49,44.7 111.76,46.43 X1.23
N$2  (via drill 0.41)
  Top 0.203: v52.63,32.11 52.32,32.41 35.76,32.41 v35.26,32.92
  Bottom 0.203: v52.63,32.11 52.63,31.19 52.73,31.09 IC3.13 | v35.26,32.92 35.05,32.72 35.05,31.9 34.95,31.8 R30.2
N$3  (via drill 0.41)
  Top 0.203: v31.5,26.52 21.13,26.52 21.13,28.85 18.59,31.39 12.8,31.39 12.8,35.05 11.99,35.87 10.16,35.87 9.45,36.58 JP5.4 | v37.08,26.52 38,27.43 v39.32,27.43 | v47.14,33.43 48.56,34.85 53.03,34.85 53.24,34.65 v54.76,34.65 | v55.68,38.1 55.98,38.41 60.76,38.41 61.67,39.32 JP3.4
  Bottom 0.203: v37.08,26.52 v31.5,26.52 | v39.32,27.43 43.48,31.6 43.48,32 43.89,32.41 46.53,32.41 46.53,32.82 v47.14,33.43 | v54.76,34.65 55.68,35.56 v55.68,38.1
N$4  (via drill 0.41)
  Top 0.203: v95.71,56.29 97.74,54.25 103.83,54.25 109.12,48.97 110.44,48.97 111.86,47.55 113.08,47.55 115.32,45.31 115.32,3.35 88.29,3.35 87.27,4.37 K1.16
  Bottom 0.203: v95.71,56.29 93.78,58.22 IC1.18
N$5  (via drill 0.41)
  Top 0.203: v66.34,68.68 66.55,68.48 83.92,68.48 v85.45,66.95
  Bottom 0.203: v66.34,68.68 66.34,68.38 67.16,68.38 IC2.1 | v85.45,66.95 86.06,66.34 86.06,60.15 84.23,58.32 83.72,58.32 IC1.1
N$6
  Top 0.305: K2.S1 94.89,16.05 97.13,18.29 105.56,18.29 109.12,21.84 110.34,21.84 111.76,23.27 112.27,23.27 114.4,25.4 114.4,43.69 111.76,43.69 X1.22
N$7
  Bottom 0.203: R4.1 13.31,38.91 11.48,38.91 11.48,39.62 U$7.A2
N$8  (via drill 0.41)
  Top 0.203: v19.51,35.46 19.51,35.87 17.37,38 16.15,38 15.75,38.41 10.87,38.41 10.36,37.9 8.03,37.9 8.03,35.46 9.35,34.14 JP5.5 | v21.13,35.46 22.15,36.47 v32.21,36.47 | v33.63,37.9 33.83,37.69 51.61,37.69 52.53,36.78 56.29,36.78 56.49,36.98 61.57,36.98 61.67,36.88 JP3.5
  Bottom 0.203: v21.13,35.46 v19.51,35.46 | v33.63,37.9 v32.21,36.47
N$9  (via drill 0.41)
  Top 0.203: v87.38,53.54 v92.15,58.32 | v88.8,32.72 v85.65,35.87
  Bottom 0.203: v92.15,58.32 92.15,59.54 93.67,59.54 IC1.17 | v87.38,53.54 85.65,51.82 v85.65,35.87 | v88.8,32.72 88.49,32.41 88.49,19.71 88.09,19.3 88.09,11.79 87.27,10.97 K2.16
N$10
  Top 0.305: K3.S1 94.89,22.55 96.93,24.59 110.34,24.59 111.76,26.01 112.27,26.01 113.89,27.64 113.89,40.95 111.76,40.95 X1.21
N$11
  Bottom 0.203: R3.1 13.31,35.26 11.48,35.26 11.48,34.65 U$7.A3
N$12  (via drill 0.41)
  Top 0.203: v15.85,44.4 16.15,44.7 19.41,44.7 v22.35,47.65 | v22.86,60.15 23.98,61.27 51,61.27 51.31,61.57 60.45,61.57 v61.77,60.25
  Bottom 0.203: v15.85,44.4 15.85,44.2 13.61,41.96 13.61,41.76 9.45,41.76 JP5.2 | v22.35,47.65 22.66,47.95 22.66,54.56 22.86,54.76 v22.86,60.15 | v61.77,60.25 60.45,58.93 60.45,45.72 61.67,44.5 JP3.2
N$13  (via drill 0.41)
  Top 0.203: v95.3,57.71 93.47,55.88 93.47,50.9 v91.75,50.9 | v89.1,19.3 87.27,17.48 K3.16
  Bottom 0.203: v95.3,57.71 95.3,60.76 93.78,60.76 IC1.16 | v91.75,50.9 91.34,50.49 91.34,21.54 v89.1,19.3
N$14
  Top 0.305: X1.20 112.88,38.2 112.88,34.95 112.27,34.34 111.76,34.34 110.34,32.92 109.22,32.92 105.66,29.36 95.2,29.36 94.89,29.06 K4.S1
N$17  (via drill 0.41)
  Top 0.203: v93.47,41.25 92.05,39.83 v88.8,39.83
  Bottom 0.203: v93.47,41.25 93.47,43.38 96.42,46.33 96.42,62.08 93.78,62.08 IC1.15 | v88.8,39.83 88.09,39.12 88.09,24.79 87.27,23.98 K4.16
N$18
  Top 0.305: X1.19 94.89,35.46 K5.S1
N$19  (via drill 0.41)
  Top 0.203: v49.17,36.98 48.97,37.19 v23.06,37.19
  Bottom 0.203: v49.17,36.98 49.17,34.54 52.02,31.7 52.02,31.19 52.12,31.09 IC3.12 | v23.06,37.19 22.55,36.68 22.55,32.11 22.25,31.8 R31.2
N$21  (via drill 0.41)
  Top 0.203: v95.4,63.3 93.07,60.96 v90.63,60.96 | v89.2,30.89 88.8,30.48 87.27,30.48 K5.16
  Bottom 0.203: v95.4,63.3 93.78,63.3 IC1.14 | v90.63,60.96 89.51,59.84 89.51,31.19 v89.2,30.89
N$22  (via drill 0.3)
  Top 0.305: v112.06,36.78 111.56,36.78 110.34,38 109.22,38 105.56,41.66 95.2,41.66 94.89,41.96 K6.S1
  Bottom 0.305: v112.06,36.78 112.88,35.97 112.88,33.83 111.76,32.72 X1.18
N$23  (via drill 0.41)
  Top 0.203: v50.39,28.25 49.58,29.06 49.58,30.89 71.93,30.89 72.24,31.19 79.45,31.19 v80.87,29.77
  Bottom 0.203: v50.39,28.25 51.71,29.57 51.71,30.28 51.61,30.38 51.61,30.89 51.51,30.99 IC3.11 | v80.87,29.77 84.63,26.01 84.63,16.26 R32.2
N$25  (via drill 0.41)
  Top 0.203: v88.8,56.9 v92.15,60.25
  Bottom 0.203: v92.15,60.25 92.15,64.62 93.67,64.62 IC1.13 | v88.8,56.9 88.49,56.59 88.49,40.54 87.27,39.32 87.27,36.98 K6.16
N$26  (via drill 0.3)
  Top 0.305: v103.12,53.65 96.22,53.65 94.89,54.97 K7.S1
  Bottom 0.305: v103.12,53.65 108.1,48.67 108.1,41.86 109.22,40.74 110.64,40.74 110.64,31.09 111.76,29.97 X1.17
N$29  (via drill 0.41)
  Top 0.203: v91.34,51.92 90.32,50.9 88.19,50.9 87.27,49.99 K7.16
  Bottom 0.203: v91.34,51.92 91.34,65.84 93.67,65.84 IC1.12
N$30  (via drill 0.3)
  Top 0.305: v97.43,43.18 v94.89,45.72 | v100.48,27.23 111.76,27.23 X1.16
  Bottom 0.305: v94.89,45.72 94.89,48.46 K8.S1 | v97.43,43.18 97.43,30.28 v100.48,27.23
N$31  (via drill 0.41)
  Top 0.203: v51,29.97 51.51,30.48 v72.54,30.48
  Bottom 0.203: v51,29.97 51,30.89 50.9,30.99 IC3.10 | v72.54,30.48 72.34,30.28 72.34,16.15 R33.2
N$33
  Bottom 0.203: IC1.11 93.67,67.16 88.09,67.16 88.09,44.3 87.27,43.48 K8.16
N$34  (via drill 0.41)
  Top 0.203: v67.87,64.01 71.22,60.66 75.89,60.66 78.03,58.52 v82.09,58.52
  Bottom 0.203: v67.87,64.01 67.87,68.28 IC2.2 | v82.09,58.52 83.11,59.54 83.62,59.54 IC1.2
N$35  (via drill 0.41)
  Top 0.203: v66.65,69.6 67.36,68.89 84.63,68.89 86.16,67.36 86.16,61.98 v85.34,61.98
  Bottom 0.203: v66.65,69.6 67.97,69.6 68.38,69.19 68.38,68.38 IC2.3 | v85.34,61.98 84.23,60.86 83.72,60.86 IC1.3
N$36  (via drill 0.41)
  Top 0.203: v68.99,66.04 66.04,66.04 65.53,66.55 65.53,67.77 v76.4,67.77
  Bottom 0.203: v68.99,66.04 68.99,68.17 69.09,68.28 IC2.4 | v76.4,67.77 81.99,62.18 83.62,62.18 IC1.4
N$37  (via drill 0.41)
  Top 0.203: v69.9,65.23 72.03,63.09 v82.09,63.09
  Bottom 0.203: v69.9,65.23 69.9,68.17 69.8,68.28 IC2.5 | v82.09,63.09 83.62,63.09 83.62,63.3 IC1.5
N$38  (via drill 0.41)
  Top 0.203: v71.42,64.72 71.63,64.52 v82.09,64.52
  Bottom 0.203: v71.42,64.72 70.41,65.73 70.41,68.28 IC2.6 | v82.09,64.52 83.62,64.52 83.62,64.62 IC1.6
N$39  (via drill 0.41)
  Top 0.203: v71.12,66.04 71.83,65.33 v81.58,65.33
  Bottom 0.203: v71.12,66.04 71.12,68.28 IC2.7 | v81.58,65.33 83.62,65.33 83.62,65.84 IC1.7
N$40  (via drill 0.41)
  Top 0.203: v85.34,66.04 v72.34,66.04
  Bottom 0.203: v72.34,66.04 71.83,66.55 71.83,68.17 71.73,68.28 IC2.8 | v85.34,66.04 84.23,67.16 83.72,67.16 IC1.8
N$45  (via drill 0.41)
  Top 0.203: v23.98,15.65 13.51,15.65 8.33,20.83 6.81,20.83 6.81,30.18 7.62,30.99 8.84,30.99 9.35,31.5 JP5.6 | v23.98,12.09 27.13,8.94 v42.67,8.94 | v50.9,20.22 51.21,19.91 59.33,19.91 60.45,21.03 v61.16,21.03
  Bottom 0.203: v23.98,12.09 v23.98,15.65 | v42.67,8.94 48.77,15.04 48.77,18.09 v50.9,20.22 | v61.16,21.03 61.77,21.64 61.77,34.24 JP3.6
N$47
  Bottom 0.203: R13.2 69.8,9.04 71.83,9.04 71.83,9.14 OK1.3
N$48
  Bottom 0.203: R14.2 69.9,4.17 71.83,4.17 OK1.1
N$49  (via drill 0.3)
  Top 0.152: v79.45,6.6 80.67,5.38 97.84,5.38 99.47,3.76 104.95,3.76 114.91,13.72 114.91,45.11 X1.10
  Bottom 0.152: v79.45,6.6 71.93,6.6 OK1.2
N$50
  Bottom 0.203: R15.2 54.56,4.17 56.39,4.17 OK2.1
N$51
  Bottom 0.203: IC2.21 71.73,61.06 71.83,60.96 71.83,51.31 74.07,49.07 74.07,12.9 80.06,6.91 80.06,5.49 81.38,4.17 OK1.8
N$52
  Bottom 0.203: R16.2 54.56,9.04 56.39,9.04 56.39,9.14 OK2.3
N$53
  Bottom 0.203: R17.2 39.12,4.17 40.95,4.17 OK3.1
N$54
  Bottom 0.203: R18.2 39.12,9.25 40.95,9.25 OK3.3
N$55  (via drill 0.3)
  Top 0.152: v47.65,6.71 49.99,9.04 86.46,9.04 86.87,8.64 92.96,8.64 v93.67,9.35 | v96.72,32.61 96.93,32.41 107.59,32.41 109.22,34.04 X1.6
  Bottom 0.152: v47.65,6.71 41.05,6.71 OK3.2 | v93.67,9.35 93.88,9.55 93.88,26.92 96.72,29.77 v96.72,32.61
N$56
  Bottom 0.203: R19.2 23.47,4.17 25.6,4.17 OK4.1
N$57
  Bottom 0.203: R20.2 23.57,9.25 25.6,9.25 OK4.3
N$58  (via drill 0.41)
  Top 0.203: v50.29,29.36 51.1,28.55 v59.23,28.55
  Bottom 0.203: v50.29,29.36 50.29,30.89 50.19,30.99 IC3.9 | v59.23,28.55 59.23,18.8 59.44,18.59 59.44,16.46 59.74,16.15 R34.2
N$59  (via drill 0.41)
  Top 0.203: v46.23,23.77 v49.38,26.92
  Bottom 0.203: v49.38,26.92 49.38,30.89 49.48,30.99 IC3.8 | v46.23,23.77 47.24,22.76 47.24,16.15 R35.2
N$60  (via drill 0.3)
  Top 0.152: v73.46,26.72 74.47,27.74 100.08,27.74 101.19,28.85 108,28.85 109.42,30.28 110.64,30.28 111.96,31.6 112.17,31.6 113.39,32.82 113.39,39.93 111.25,39.93 109.22,41.96 X1.9
  Bottom 0.152: v73.46,26.72 73.46,13.31 71.93,11.79 OK1.4
N$61  (via drill 0.3)
  Top 0.152: v62.48,6.71 63.2,7.42 92.56,7.42 93.57,8.43 v94.89,8.43
  Bottom 0.152: v62.48,6.71 56.49,6.71 OK2.2 | v94.89,8.43 97.84,11.38 97.84,21.95 104.85,28.96 106.88,28.96 106.88,37.19 109.22,39.52 X1.8
N$62  (via drill 0.3)
  Top 0.152: v61.37,13.61 63.3,15.54 86.46,15.54 86.87,15.14 98.04,15.14 100.69,17.78 v106.58,17.78
  Bottom 0.152: v61.37,13.61 61.37,11.79 56.49,11.79 OK2.4 | v106.58,17.78 107.19,18.39 107.19,28.75 108.1,29.67 108.1,35.66 109.22,36.78 X1.7
N$63  (via drill 0.41)
  Top 0.203: v66.34,58.62 65.02,57.3 v50.19,57.3 | v34.34,44.09 v41.55,44.09 | v34.34,32.92 34.34,30.48 v38.91,30.48 | v36.88,14.94 35.87,13.92 v35.05,13.92
  Bottom 0.203: v66.34,58.62 66.85,59.13 66.85,60.76 67.16,61.06 IC2.28 | v50.19,57.3 47.04,54.15 47.04,49.58 v41.55,44.09 | v34.34,32.92 v34.34,44.09 | v38.91,30.48 38.61,30.18 38.61,23.27 36.58,21.23 36.58,16.97 36.88,16.66 v36.88,14.94 | v35.05,13.92 33.83,12.7 33.83,10.46 35.05,9.25 OK4.6
N$64  (via drill 0.3)
  Top 0.152: v42.47,13.21 42.67,13.01 103.94,13.01 v104.24,13.31
  Bottom 0.152: v42.47,13.21 41.05,11.79 OK3.4 | v104.24,13.31 107.59,13.31 107.59,28.45 109.22,30.07 X1.5
N$65  (via drill 0.3)
  Top 0.152: v28.75,10.26 30.68,12.19 104.95,12.19 v112.78,20.02
  Bottom 0.152: v28.75,10.26 28.75,9.75 25.7,6.71 OK4.2 | v112.78,20.02 112.88,20.12 112.88,27.53 111.56,28.85 109.22,28.85 X1.4
N$66  (via drill 0.3)
  Top 0.152: v27.23,11.79 28.04,12.6 104.44,12.6 v108.31,16.46
  Bottom 0.152: v27.23,11.79 25.7,11.79 OK4.4 | v108.31,16.46 108.1,16.66 108.1,24.59 109.22,25.7 X1.3
N$67
  Bottom 0.203: IC3.7 48.87,31.09 48.77,31.19 48.77,36.37 48.16,36.98 38.2,36.98 38.2,24.89 35.66,22.35 35.66,20.22 34.04,18.59 34.04,16.87 34.75,16.15 R36.2
N$68  (via drill 0.41)
  Top 0.203: v73.25,27.74 72.34,26.82 v71.12,26.82 | v71.12,25.4 71.53,24.99 v74.78,24.99
  Bottom 0.203: v73.25,27.74 73.25,49.28 71.12,51.41 71.12,61.06 IC2.22 | v71.12,25.4 v71.12,26.82 | v74.78,24.99 75.29,24.49 75.29,14.63 80.67,9.25 81.38,9.25 OK1.6
N$69  (via drill 0.41)
  Top 0.203: v70.41,55.17 72.95,52.63 75.89,52.63 77.32,54.05 v78.33,54.05 | v82.3,57.51 v80.37,57.51 | v86.26,57.51 87.58,56.19 89.1,56.19 91.44,58.52 91.44,58.93 91.75,58.93 91.85,59.03 99.67,59.03 106.98,51.71 110.54,51.71 111.86,50.39 v112.57,50.39 | v67.67,3.56 v83.01,3.56
  Bottom 0.203: v70.41,55.17 70.41,61.06 IC2.23 | v78.33,54.05 80.37,56.08 v80.37,57.51 | v86.26,57.51 v82.3,57.51 | v112.57,50.39 114,48.97 114,10.16 107.39,3.56 v83.01,3.56 | v67.67,3.56 66.04,3.56 66.04,4.06 OK2.8
N$70  (via drill 0.41)
  Top 0.203: v71.73,49.78 v68.99,52.53 | v72.54,34.04 70.51,32 v67.56,32
  Bottom 0.203: v68.99,52.53 68.99,57.3 69.39,57.71 69.39,59.84 69.7,60.15 69.7,61.06 IC2.24 | v71.73,49.78 72.54,48.97 v72.54,34.04 | v67.56,32 66.55,30.99 66.55,25.09 63.4,21.95 63.4,21.03 64.52,19.91 64.52,16.05 63.4,14.94 63.4,11.79 65.94,9.25 OK2.6
N$71  (via drill 0.41)
  Top 0.203: v65.23,55.47 v67.46,55.47 | v59.13,13.72 59.13,15.65 55.27,15.65 v55.07,15.44 | v57,20.62 57.2,20.42 59.23,20.42 60.76,21.95 v61.06,21.95 | v61.06,32 58.22,34.85 v57.2,34.85 | v58.12,39.12 59.23,40.23 v59.23,41.86 | v59.23,46.94 59.23,48.97 v63.6,48.97
  Bottom 0.203: v67.46,55.47 68.38,56.39 68.38,59.33 68.99,59.94 68.99,60.96 69.09,61.06 IC2.25 | v65.23,55.47 63.6,53.85 v63.6,48.97 63.6,44.7 63.91,44.4 | v59.13,13.72 59.13,13.41 55.88,13.41 53.65,11.18 53.65,7.21 50.6,4.17 OK3.8 | v55.07,15.44 56.9,17.27 56.9,20.52 v57,20.62 | v61.06,32 v61.06,21.95 | v57.2,34.85 56.08,35.97 56.08,37.08 v58.12,39.12 | v59.23,46.94 v59.23,41.86
N$72  (via drill 0.41)
  Top 0.203: v67.67,57.61 66.65,56.59 43.99,56.59 43.08,55.68 v21.34,55.68 | v21.84,27.23 v21.84,32.92 | v24.99,13.11 28.45,9.65 v48.97,9.65
  Bottom 0.203: v67.67,57.61 67.67,59.33 68.38,60.05 68.38,61.06 IC2.26 | v21.34,55.68 21.34,41.25 21.84,40.74 v21.84,32.92 | v21.84,27.23 24.99,24.08 v24.99,13.11 | v48.97,9.65 50.49,9.65 50.49,9.25 OK3.6
N$73  (via drill 0.41)
  Top 0.203: v46.63,54.76 v66.85,54.76 | v38.51,39.62 38.3,39.42 21.44,39.42 20.22,38.2 20.22,34.65 v23.27,34.65
  Bottom 0.203: v66.85,54.76 66.75,54.86 66.75,57.71 67.26,58.22 67.26,59.54 67.77,60.05 67.77,61.06 IC2.27 | v46.63,54.76 46.63,50.19 38.41,41.96 38.41,39.73 v38.51,39.62 | v23.27,34.65 25.5,32.41 25.5,14.43 33.83,6.1 33.83,5.38 35.05,4.17 OK4.8
N$74  (via drill 0.41)
  Top 0.203: v48.16,29.97 47.95,29.77 35.76,29.77 29.26,23.27 v24.28,23.27
  Bottom 0.203: v48.16,29.97 48.16,30.99 IC3.6 | v24.28,23.27 22.35,21.34 22.35,16.66 22.25,16.56 R37.2
N$75  (via drill 0.41)
  Top 0.203: v54.25,25.3 54.36,25.4 v57,25.4 | v47.85,36.27 v56.79,36.27
  Bottom 0.203: v54.25,25.3 53.44,25.3 IC3.15 | v57,25.4 58.52,26.92 58.52,30.79 59.13,31.39 59.13,33.93 v56.79,36.27 | v47.85,36.27 47.35,35.76 47.35,35.15 R29.2
N$76  (via drill 0.41)
  Top 0.203: v52.93,29.26 53.44,29.77 v56.59,29.77
  Bottom 0.203: v52.93,29.26 52.93,25.4 52.83,25.3 IC3.16 | v56.59,29.77 56.39,29.97 56.39,31.8 R28.2
N$77  (via drill 0.41)
  Top 0.203: v52.22,26.82 53.34,27.94 58.83,27.94 59.03,27.74 v67.67,27.74
  Bottom 0.203: v52.22,26.82 52.22,25.3 IC3.17 | v67.67,27.74 68.68,28.75 68.68,31.7 R27.2
N$78  (via drill 0.41)
  Top 0.203: v55.37,23.57 55.88,23.06 v78.54,23.06
  Bottom 0.203: v55.37,23.57 52.63,23.57 51.61,24.59 51.61,25.09 51.51,25.2 IC3.18 | v78.54,23.06 80.16,24.69 80.16,30.58 81.28,31.7 R26.2
N$79  (via drill 0.41)
  Top 0.203: v51,22.66 74.27,22.66 76.5,20.42 90.63,20.42 91.85,21.64 96.93,21.64 99.16,23.88 v104.04,23.88
  Bottom 0.203: v51,22.66 51,25.09 50.9,25.2 IC3.19 | v104.04,23.88 105.97,21.95 105.97,17.88 104.95,16.87 R25.2
N$80  (via drill 0.41)
  Top 0.203: v50.29,26.82 51,26.11 76.4,26.11 76.5,26.01 v100.28,26.01
  Bottom 0.203: v50.29,26.82 50.29,25.4 50.19,25.3 IC3.20 | v100.28,26.01 104.04,29.77 R24.2
N$81  (via drill 0.41)
  Top 0.203: v49.89,22.05 48.26,20.42 40.84,20.42 40.74,20.52 40.03,20.52 39.93,20.42 35.26,20.42 v34.95,20.73
  Bottom 0.203: v49.89,22.05 49.68,22.25 49.68,25.09 49.58,25.2 IC3.21 | v34.95,20.73 35.26,21.03 35.26,23.16 37.8,25.7 37.8,44.81 43.69,50.7 R23.2
N$82  (via drill 0.41)
  Top 0.203: v49.17,20.02 49.68,19.51 v59.94,19.51
  Bottom 0.203: v49.17,20.02 49.17,23.27 49.07,23.37 49.07,25.09 48.97,25.2 IC3.22 | v59.94,19.51 59.64,19.81 59.64,27.94 59.94,28.25 59.94,47.24 56.39,50.8 R22.2
RES  (via drill 0.41)
  Top 0.203: RESETA.3 13.21,6.4 15.75,6.4 RESET.3 | v30.58,15.85 30.38,15.65 24.99,15.65 v19,9.65
  Bottom 0.203: v30.58,15.85 32.72,17.98 GND.RES | v19,9.65 15.75,6.4 RESET.3
SDI_MOSI  (via drill 0.41)
  Top 0.203: v74.78,34.14 76.91,32 100.08,32 101.3,30.79 JP2.2
  Bottom 0.203: v74.78,34.14 74.78,46.13 76,47.35 SERIAL.8
SDI_SCLK  (via drill 0.41)
  Top 0.203: v75.89,32 76.3,31.6 97.94,31.6 98.75,30.79 JP2.1
  Bottom 0.203: v75.89,32 75.89,44.7 76,44.81 SERIAL.7
SLIDER_IN  (via drill 0.41)
  Top 0.203: v52.73,15.85 53.03,16.15 63.09,16.15 63.7,16.76 65.13,16.76 v65.23,16.87 | v71.83,40.23 75.08,43.48 77.22,43.48 78.54,44.81 SERIAL.5
  Bottom 0.203: C7.1 75.79,55.68 73.66,55.68 73.66,54.36 POT1.2A 73.66,54.25 75.79,52.12 75.79,49.48 77.32,47.95 77.32,46.13 78.54,44.91 SERIAL.5 | v52.73,15.85 50.6,17.98 GND.A0 | v65.23,16.87 68.78,20.42 71.83,20.42 v71.83,40.23

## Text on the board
_tsilk: SCL SDA
_bsilk: SKAARHOJ 2013 | PCB-CMB-5-SHLD v09-13/2 | I2C PullUps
